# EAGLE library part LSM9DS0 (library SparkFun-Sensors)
LSM9DS0 3D Accelerometer, 3D Gyroscope, 3D Magnetomter Replaced by LSM9DS1 Features: 3 acceleration channels, 3 angular rate channels, 3 magnetic field channels ±2/±4/±6/±8/±16 g linear acceleration full scale ±2/±4/±8/±12 gauss magnetic full scale ±245/±500/±2000 dps angular rate full scale 16-bit data output SPI / I2C serial interfaces Analog supply voltage 2.4 V to 3.6 V Power-down mode / low-power mode Programmable interrupt generators Embedded self-test Embedded temperature sensor Embedded FIFO Position and motion detection functions Click/double-click recognition Datasheet SparkFun Products SparkFun Block for Intel® Edison - 9 Degrees of Freedom (DEV-13033)
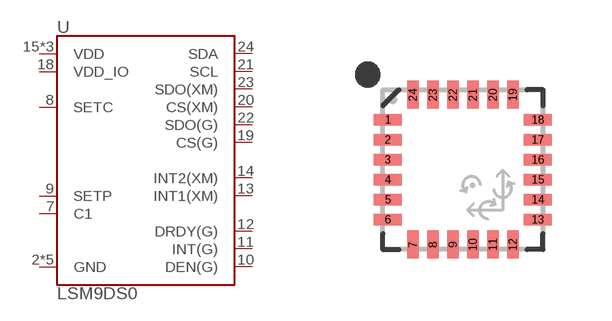
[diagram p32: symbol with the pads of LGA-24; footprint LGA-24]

Designator prefix U

## LSM9DS0 (PROD_ID: IC-11867; VALUE: LSM9DS0)  [LGA-24]
2  GND
3  GND
4  GND
5  GND
6  GND
7  C1
8  SETC
9  SETP
10  DEN(G)
11  INT(G)
12  DRDY(G)
13  INT1(XM)
14  INT2(XM)
15  VDD
16  VDD
17  VDD
18  VDD_IO
19  CS(G)
20  CS(XM)
21  SCL
22  SDO(G)
23  SDO(XM)
24  SDA

## Footprint LGA-24 (pad centres in mm)
LGA 4x4x1 mm 24-lead 0.5mm pitch Pads are 0.35x0.2 mm square This package is used for: ST Micro LSM9DS0 3D accel/gyro/mag
smd 0.7 x 0.29: 1 -1.875,1.25; 2 -1.875,0.75; 3 -1.875,0.25; 4 -1.875,-0.25; 5 -1.875,-0.75; 6 -1.875,-1.25; 13 1.875,-1.25; 14 1.875,-0.75; 15 1.875,-0.25; 16 1.875,0.25; 17 1.875,0.75; 18 1.875,1.25
smd 0.29 x 0.7: 7 -1.25,-1.875; 8 -0.75,-1.875; 9 -0.25,-1.875; 10 0.25,-1.875; 11 0.75,-1.875; 12 1.25,-1.875; 19 1.25,1.875; 20 0.75,1.875; 21 0.25,1.875; 22 -0.25,1.875; 23 -0.75,1.875; 24 -1.25,1.875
